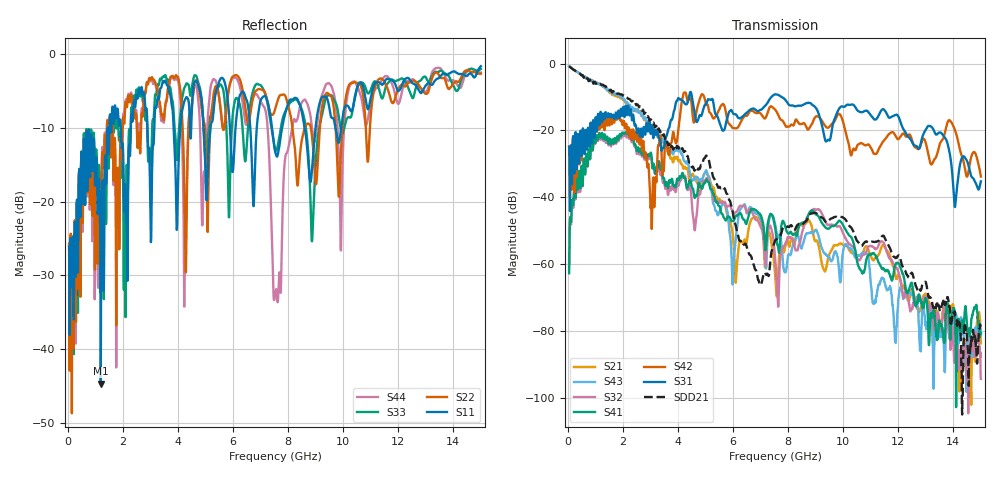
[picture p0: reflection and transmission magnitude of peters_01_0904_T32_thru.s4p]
# MHZ S RI R 50.00
! FREQ  S11  S12  S13  S14
!  S21  S22  S23  S24
!  S31  S32  S33  S34
!  S41  S42  S43  S44
!  REAL  IMAG  REAL  IMAG  REAL  IMAG  REAL  IMAG
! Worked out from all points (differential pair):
!   1496 points, 50 MHz to 15 GHz, reference 50 ohm
!   strongest paths, dB at 50 MHz, 3.79 GHz, 7.53 GHz, 11.27 GHz, 15 GHz:
!     S31: -24.9, -16.7, -9.2, -15.8, -35.3
!     S42: -24.8, -22.5, -13.8, -26.0, -33.8
!     S41: -62.7, -34.5, -49.1, -59.2, -80.8
!     S32: -60.1, -36.3, -58.3, -54.8, -94.4
!     S43: -0.8, -26.3, -48.0, -66.6, -81.1
!     S21: -0.8, -28.6, -62.9, -57.3, -83.7
!   taken as a pair (ports 3,1 in; 4,2 out), SDD21 dB: -0.8, -24.8, -53.0, -53.1, -78.3
!   lowest |S11| = -44.7 dB at 1.2 GHz (marker M1), VSWR 1.01, Z = 50.1 + j0.57 ohm
!   |S11| at or under -10 dB: start of sweep to 1.445 GHz; 7.416 GHz to 7.783 GHz (367 MHz wide, 4.83 % of centre); 8.601 GHz to 8.996 GHz (395.3 MHz wide, 4.49 % of centre)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
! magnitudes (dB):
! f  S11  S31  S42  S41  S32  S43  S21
! 50 MHz  -26.1  -24.9  -24.8  -62.7  -60.1  -0.8  -0.8
! 1.2 GHz  -44.7  -14.5  -14.9  -22.1  -22.8  -6.3  -6.4
! 3.07 GHz  -14.3  -19.1  -41.3  -30.9  -31.1  -19.4  -20.0
! 4.24 GHz  -6.3  -11.9  -8.6  -34.1  -33.7  -29.2  -31.0
! 6.11 GHz  -9.1  -15.2  -19.4  -45.5  -44.5  -51.7  -64.5
! 7.56 GHz  -13.6  -9.2  -14.1  -51.0  -61.5  -49.3  -66.7
! 15 GHz  -1.6  -35.3  -33.8  -80.8  -94.4  -81.1  -83.7
